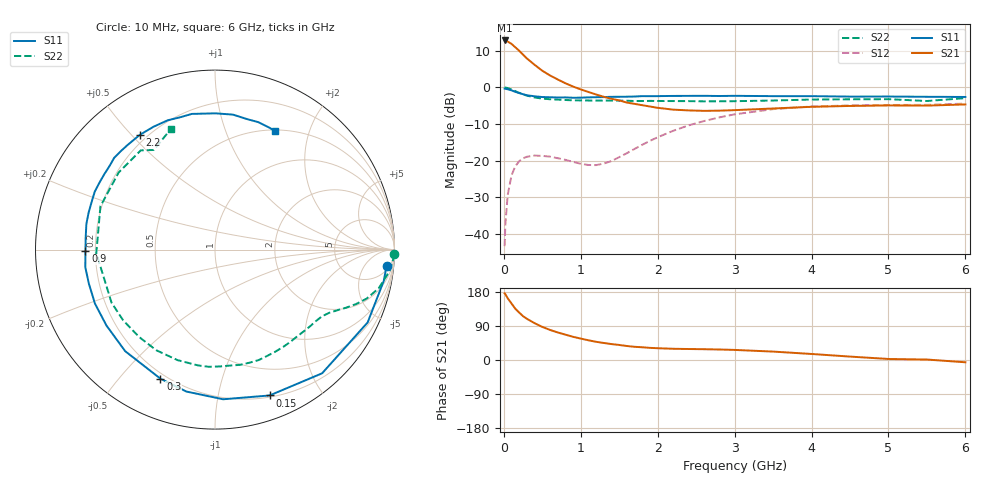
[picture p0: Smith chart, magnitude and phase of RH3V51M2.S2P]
! SIEMENS Small Signal Semiconductors
! BFR106
! Si NPN RF Bipolar Junction Transistor in SOT23
! VCE = 3.5 V  IC = 1.2 mA
! Common Emitter S-Parameters:  August  1996
# GHz  S  MA  R  50
!  f  S11  S21  S12  S22
! GHz  MAG  ANG  MAG  ANG  MAG  ANG  MAG  ANG
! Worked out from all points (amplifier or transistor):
!   36 points, 10 MHz to 6 GHz, reference 50 ohm
!   highest |S21| = 12.8 dB at 10 MHz (marker M1)
!   |S21| within 3 dB of that: start of sweep to 208.9 MHz
!   unconditionally stable (mu >= 1): 851.1 MHz to 2.032 GHz; 2.753 GHz to end of sweep
!   at 250 MHz: K = 0.27, MSG = 14.1 dB, |S12| = -19.3 dB
!   at 1.4 GHz: K = 1.38, MAG = 4.8 dB, |S12| = -20.1 dB
!   at 6 GHz: K = 1.02, MAG = -1.0 dB, |S12| = -4.4 dB
!   S11 on the Smith chart (normalised r, x): 10 MHz: 8, -18; 150 MHz: 0.22, -1.42; 300 MHz: 0.18, -0.65; 900 MHz: 0.16, -0.01; 2.2 GHz: 0.17, +0.53; 6 GHz: 0.52, +1.50
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0.01  0.9602 -5.3  4.37 176.0  0.0068 89.1  0.9999 -1.5
0.02  0.9564 -10.5  4.347 173.5  0.0135 84.3  0.9955 -2.9
0.05  0.9423 -25.5  4.225 163.0  0.0339 75.3  0.9791 -7.1
0.1  0.9117 -49.1  3.922 149.0  0.0631 63.1  0.938 -13.2
0.15  0.8677 -69.5  3.52 135.0  0.084 52.0  0.8881 -17.9
0.2  0.8351 -86.9  3.162 125.1  0.0984 44.2  0.8425 -21.1
0.25  0.8067 -101.4  2.797 115.6  0.1078 37.1  0.8004 -23.8
0.3  0.7808 -112.9  2.481 108.7  0.113 32.3  0.772 -25.6
0.4  0.7554 -131.5  2.032 97.1  0.1173 24.9  0.7278 -28.9
0.5  0.738 -145.0  1.686 87.3  0.1161 20.5  0.7021 -32.0
0.7  0.7279 -165.0  1.283 72.7  0.108 17.5  0.6807 -38.9
0.9  0.7219 -179.3  1.026 61.2  0.0962 21.5  0.6661 -46.4
1.1  0.7308 168.7  0.865 52.0  0.0872 32.8  0.6621 -54.9
1.3  0.7371 158.7  0.743 44.9  0.0913 49.5  0.6598 -63.8
1.6  0.7462 145.8  0.62 36.9  0.1265 68.1  0.657 -77.8
2.2  0.7645 123.3  0.497 29.6  0.2552 70.1  0.6502 -108.7
2.8  0.7624 104.9  0.481 27.7  0.3889 56.4  0.646 -142.4
3.5  0.7592 89.8  0.515 22.2  0.5047 38.1  0.6616 -178.3
4.5  0.7487 76.3  0.558 9.0  0.5668 15.9  0.6875 141.3
5  0.7499 71.3  0.567 2.7  0.5751 7.7  0.6904 126.8
5.5  0.7439 66.0  0.564 1.2  0.5775 3.8  0.6516 121.6
6  0.7398 63.1  0.585 -6.0  0.601 -4.0  0.7137 110.3
